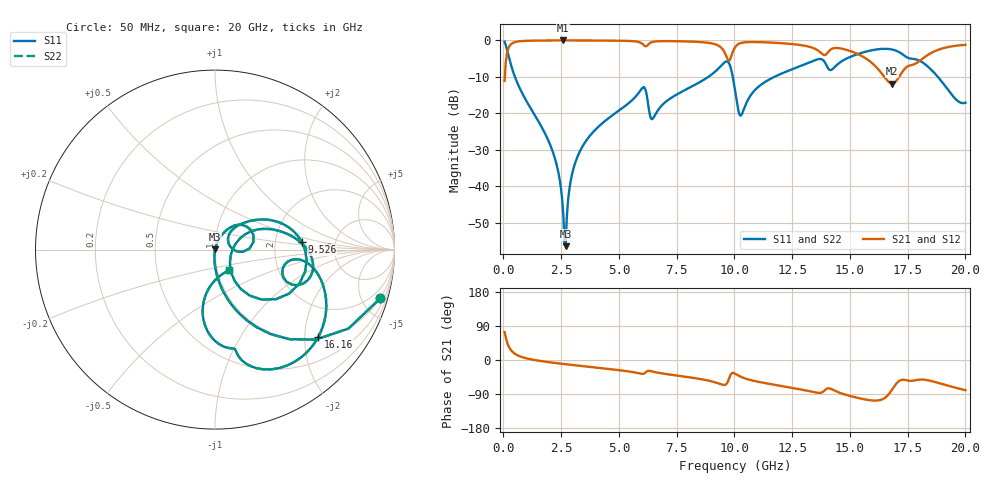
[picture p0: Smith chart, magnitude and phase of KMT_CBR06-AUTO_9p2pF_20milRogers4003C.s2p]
! Data measured by Modelithics Inc. support@modelithics.com 813-866-6335
! KEMET CBR06-AUTO 9.2pF, Pad Width= 0.851mm, Pad Length= 0.64mm, Pad Gap= 0.62mm, 20mil Rogers 4003C substrate Data, January 2022
# hz S ma R 50
! 2 Port Network Data from SP1.SP block
! freq  magS11  angS11  magS21  angS21  magS12  angS12  magS22  angS22
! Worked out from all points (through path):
!   401 points, 50 MHz to 20 GHz, reference 50 ohm
!   highest |S21| = -0.01 dB at 2.594 GHz (marker M1); lowest = -11.8 dB at 16.81 GHz (marker M2)
!   group delay of S21, straight-line fit = 13.1 ps
!   lowest |S11| = -56.3 dB at 2.693 GHz (marker M3), VSWR 1.00, Z = 50.1 + j0.0992 ohm
!   |S11| at or under -10 dB: 498.1 MHz to 8.867 GHz (8.369 GHz wide, 179 % of centre); 9.929 GHz to 11.72 GHz (1.794 GHz wide, 16.6 % of centre); 18.81 GHz to end of sweep
!   |S22| runs from -56.3 to -0.4 dB; largest |S21 - S12| = 0
!   S11 on the Smith chart (normalised r, x): 50 MHz: 0.98, -6.79; 9.526 GHz: 2.85, +0.32; 16.16 GHz: 1.04, -2.34; 20 GHz: 1.14, -0.27
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5e7  0.9601 -16.4  0.2795 73.5  0.2795 73.5  0.9601 -16.4
2.99375e8  0.493 -61.6  0.8694 28.3  0.8694 28.3  0.493 -61.6
5.4875e8  0.2876 -75.4  0.9571 14.4  0.9571 14.4  0.2876 -75.4
2.14475e9  0.02935 -95.5  0.9986 -7.2  0.9986 -7.2  0.02935 -95.5
2.444e9  0.01192 -95.0  0.9989 -9.4  0.9989 -9.4  0.01192 -95.0
2.593625e9  0.004021 -87.1  0.999 -10.5  0.999 -10.5  0.004021 -87.1
2.693375e9  0.001524 40.5  0.999 -11.2  0.999 -11.2  0.001524 40.5
2.94275e9  0.01342 72.9  0.9988 -12.9  0.9988 -12.9  0.01342 72.9
3.391625e9  0.03397 72.3  0.9982 -15.9  0.9982 -15.9  0.03397 72.3
6.035e9  0.2263 29.8  0.8877 -36.6  0.8877 -36.6  0.2263 29.8
6.434e9  0.08332 23.4  0.948 -30.1  0.948 -30.1  0.08332 23.4
6.73325e9  0.1158 47.2  0.9755 -34.0  0.9755 -34.0  0.1158 47.2
9.52625e9  0.4858 5.0  0.7281 -65.8  0.7281 -65.8  0.4858 5.0
1.0025e10  0.2091 -57.9  0.8026 -35.9  0.8026 -35.9  0.2091 -57.9
1.027438e10  0.09326 -11.7  0.9198 -44.2  0.9198 -44.2  0.09326 -11.7
1.117212e10  0.2503 25.8  0.9464 -59.2  0.9464 -59.2  0.2503 25.8
1.336662e10  0.5182 -0.6  0.7968 -84.0  0.7968 -84.0  0.5182 -0.6
1.615962e10  0.7532 -40.1  0.4249 -107.0  0.4249 -107.0  0.7532 -40.1
1.670825e10  0.762 -57.2  0.2659 -88.1  0.2659 -88.1  0.762 -57.2
1.6808e10  0.7533 -60.6  0.2566 -79.6  0.2566 -79.6  0.7533 -60.6
1.845388e10  0.4163 -98.1  0.656 -54.5  0.656 -54.5  0.4163 -98.1
2e10  0.1402 -55.6  0.8697 -79.7  0.8697 -79.7  0.1402 -55.6
